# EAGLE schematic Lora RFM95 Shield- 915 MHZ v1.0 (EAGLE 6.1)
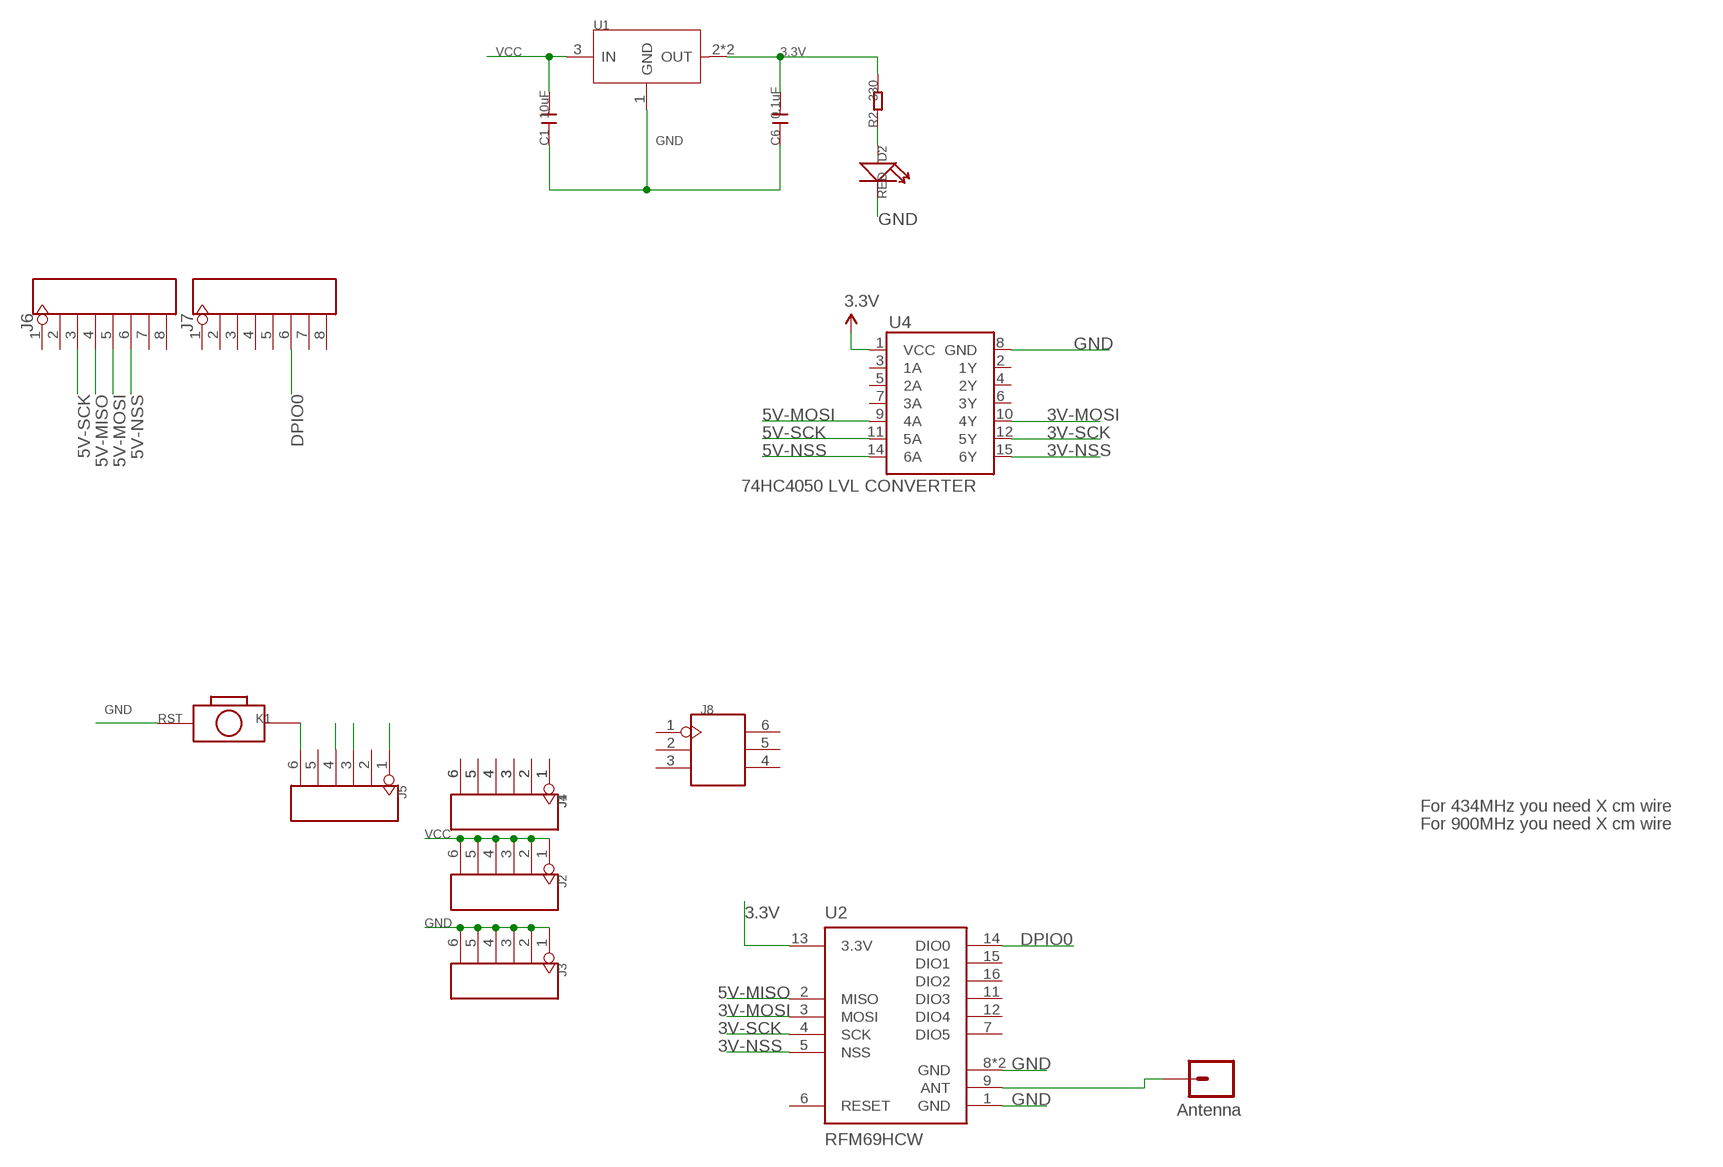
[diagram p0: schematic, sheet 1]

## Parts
ANT  Antenna  M01PTH  [1X01]
C1  10uF  C-0805  [C0805]
C6  0.1uF  C-0603  [C0603]
D2  RED  LED'0603'  [LED-0603]
J1  HEADER-6P-65/35MIL  [6P-2.54-65/35MIL]
J2  HEADER-6P-65/35MIL  [6P-2.54-65/35MIL]
J3  HEADER-6P-65/35MIL  [6P-2.54-65/35MIL]
J4  HEADER-6P-65/35MIL  [6P-2.54-65/35MIL]
J5  HEADER-6P-65/35MIL  [6P-2.54-65/35MIL]
J6  HEADER-8P-65/35MIL  [8P-2.54-65/35MIL]
J7  HEADER-8P-65/35MIL  [8P-2.54-65/35MIL]
J8  HEADER-2X3P-65/35MIL  [2X3P-2.54-65/35MIL]
R2  330  R-0603  [R0603]
RST  K1  BOTTON-2P-90D  [2P-7.62X3.56-90D]
U1  LD1117'SOT89'  [SOT89]
U2  RFM69HCW  [RFM69HCW-XXXS2]
U4  74HC4050 LVL CONVERTER  HEX_CONVERTER  [SO016]

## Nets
3.3V: C6.2 R2.2 U1.2(OUT) U1.4(OUT) U2.13(3.3V) U4.1(VCC)
3V-MOSI: U2.3(MOSI) U4.10(4Y)
3V-NSS: U2.5(NSS) U4.15(6Y)
3V-SCK: U2.4(SCK) U4.12(5Y)
5V-MISO: J6.4 U2.2(MISO)
5V-MOSI: J6.5 U4.9(4A)
5V-NSS: J6.6 U4.14(6A)
5V-SCK: J6.3 U4.11(5A)
DPIO0: J7.6 U2.14(DIO0)
GND: C1.1 C6.1 D2.- J3.1 J3.2 J3.3 J3.4 J3.5 J3.6 J5.3 RST.P$1 U1.1(GND) U2.1(GND) U2.8(GND) U2.10(GND) U4.8(GND)
N$1: ANT.1 U2.9(ANT)
N$2: D2.+ R2.1
N$7: J5.6 RST.P$2
N$10: J5.1
PC0: J1.6 J4.6
PC1: J1.5 J4.5
PC2: J1.4 J4.4
PC3: J1.3 J4.3
PC4: J1.2 J4.2
PC5: J1.1 J4.1
VCC: C1.2 J2.1 J2.2 J2.3 J2.4 J2.5 J2.6 J5.4 U1.3(IN)
Unconnected: J5.2 J5.5 J6.1 J6.2 J6.7 J6.8 J7.1 J7.2 J7.3 J7.4 J7.5 J7.7 J7.8 J8.1 J8.2 J8.3 J8.4 J8.5 J8.6 U2.6(RESET) U2.7(DIO5) U2.11(DIO3) U2.12(DIO4) U2.15(DIO1) U2.16(DIO2) U4.2(1Y) U4.3(1A) U4.4(2Y) U4.5(2A) U4.6(3Y) U4.7(3A)

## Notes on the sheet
- For 434MHz you need X cm wire
- For 900MHz you need X cm wire

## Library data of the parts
ANT = SparkFun:M01: Header 1
C1 C6 = Discrete:C*: Ceramic Capacitors
D2 = Discrete:LED*
J1-J5 = Connector:HEADER-6P
J6 J7 = Connector:HEADER-8P
J8 = Connector:HEADER-2X3P
R2 = Discrete:R*
RST = Discrete:BOTTON-2P
U1 = IC:LD1117: Low Drop Fixed And Adjustable Positive Voltage Regulators http://www.datasheetcatalog.org/datasheet/SGSThomsonMicroelectronics/mXuqtqv.pdf
U2 = mike-temp:RFM69H
U4 = SparkFun:HEX_CONVERTER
